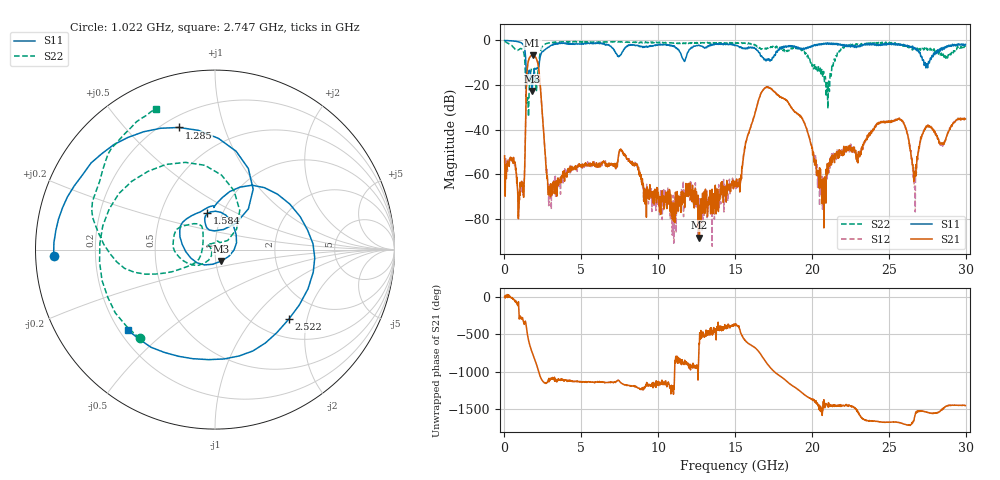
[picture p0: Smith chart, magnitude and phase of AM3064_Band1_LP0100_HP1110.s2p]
# Hz S DB R 50.0
!freq dBS11 angS11 dBS21 angS21 dBS12 angS12 dBS22 angS22
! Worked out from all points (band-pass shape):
!   1600 points, 10 MHz to 29.98 GHz, reference 50 ohm
!   highest |S21| = -6.70 dB at 1.828 GHz (marker M1); lowest = -88.4 dB at 12.68 GHz (marker M2)
!   |S21| within 3 dB of the highest: 1.543 GHz to 2.15 GHz (607.3 MHz wide, 32.9 % of centre)
!   lowest |S11| = -22.8 dB at 1.791 GHz (marker M3), VSWR 1.16, Z = 53.2 - j6.83 ohm
!   |S11| at or under -10 dB: 1.393 GHz to 2.271 GHz (878.1 MHz wide, 47.9 % of centre); 27.28125 GHz to 27.3542 GHz (72.94 MHz wide, 0.267 % of centre); 27.36 GHz to 27.57 GHz (210 MHz wide, 0.765 % of centre)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
!   |S22| runs from -34.2 to -0.5 dB; largest |S21 - S12| = 0.0093
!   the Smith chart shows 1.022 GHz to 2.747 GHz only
!   S11 on the Smith chart (normalised r, x): 1.022 GHz: 0.05, -0.02; 1.285 GHz: 0.26, +0.71; 1.584 GHz: 0.85, +0.36; 2.522 GHz: 1.37, -1.56; 2.747 GHz: 0.23, -0.37
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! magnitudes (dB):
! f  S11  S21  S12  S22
! 10 MHz  0.0  -51.8  -54.5  -0.5
! 1.022 GHz  -0.9  -63.7  -65.3  -3.8
! 1.285 GHz  -3.0  -63.5  -64.1  -6.5
! 1.584 GHz  -13.7  -8.5  -8.5  -28.3
! 1.791 GHz  -22.8  -6.7  -6.7  -12.6
! 1.828 GHz  -19.7  -6.7  -6.7  -12.4
! 2.184 GHz  -12.6  -10.7  -10.7  -13.7
! 2.522 GHz  -5.0  -38.5  -38.5  -2.3
! 2.747 GHz  -3.6  -59.3  -57.7  -1.4
! 5.015 GHz  -1.4  -56.1  -55.8  -0.8
! 7.601 GHz  -6.1  -49.8  -49.5  -0.7
! 10 GHz  -2.0  -68.4  -67.9  -1.0
! 12.68 GHz  -2.3  -88.4  -77.0  -1.1
! 15 GHz  -2.2  -64.8  -64.4  -1.4
! 17.01 GHz  -9.2  -21.2  -21.0  -3.7
! 19.99 GHz  -3.0  -47.7  -47.8  -10.8
! 20.76 GHz  -1.3  -68.1  -64.2  -13.9
! 25 GHz  -1.4  -36.1  -36.2  -1.2
! 25.99 GHz  -2.1  -37.6  -37.0  -2.3
! 26.66 GHz  -3.3  -60.7  -66.0  -4.0
! 27.39 GHz  -11.3  -39.4  -38.8  -4.3
! 29.98 GHz  -1.8  -35.2  -35.2  -2.9
